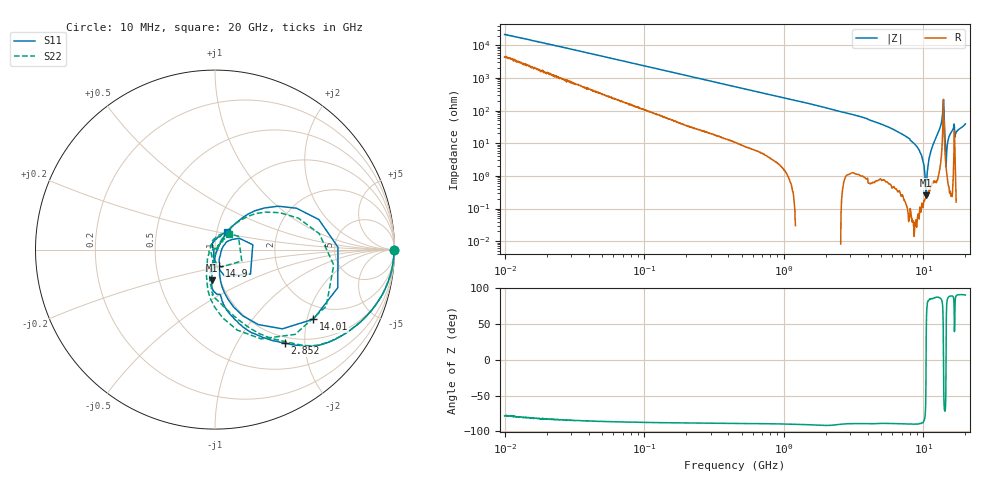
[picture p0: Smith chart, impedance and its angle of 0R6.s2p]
!Keysight Technologies,P5008B,MY61100088,A.16.20.02
!Date: Monday, October 30, 2023 15:55:42
!Correction: S11(C  2-Port  )
!S21(C  2-Port  )
!S12(C  2-Port  )
!S22(C  2-Port  )
!S2P File: Measurements: S11, S21, S12, S22:Log Frequency Sweep
# Hz S  dB  R 50
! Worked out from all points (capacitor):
!   1601 points, 10 MHz to 20 GHz, reference 50 ohm
!   read as one part in series: C = 733 fF near 10.39 MHz
!   lowest |Z| = 253 mohm at 10.43 GHz (marker M1)
!   series resonance near 10.46 GHz, so ESL is about 320 pH
!   S11 on the Smith chart (normalised r, x): 10 MHz: open; 2.852 GHz: 0.90, -1.62; 14.01 GHz: 1.55, -2.19; 14.9 GHz: 1.03, -0.19; 20 GHz: 1.12, +0.22
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1e7  -0.00 -0.3  -46.66 78.1  -46.69 78.9  -0.01 -0.3
3.555162e7  -0.01 -0.9  -36.19 84.1  -36.20 84.3  -0.01 -0.9
1.263918e8  -0.03 -3.2  -25.49 84.5  -25.49 84.5  -0.03 -3.2
4.472136e8  -0.18 -11.0  -14.84 77.8  -14.84 77.9  -0.18 -11.0
1.589917e9  -1.41 -34.7  -5.41 56.2  -5.41 56.2  -1.42 -34.6
2.851944e9  -3.73 -53.2  -2.52 36.7  -2.53 36.7  -3.76 -52.4
5.652411e9  -8.76 -77.3  -0.65 12.1  -0.65 12.1  -8.78 -76.4
1.043228e10  -15.27 -96.1  -0.12 -9.9  -0.12 -9.8  -15.18 -99.7
1.147208e10  -19.32 -96.9  -0.06 -14.1  -0.07 -14.1  -19.07 -101.7
1.214507e10  -27.15 -90.8  -0.03 -17.5  -0.03 -17.4  -27.01 -95.8
1.2437e10  -37.85 -34.3  -0.02 -19.4  -0.03 -19.4  -40.60 -46.6
1.27966e10  -25.10 51.6  -0.06 -22.4  -0.07 -22.4  -25.44 55.6
1.329228e10  -14.89 52.2  -0.32 -29.2  -0.33 -29.2  -15.20 52.8
1.361179e10  -8.85 40.0  -1.21 -39.5  -1.21 -39.5  -9.07 36.5
1.400536e10  -3.46 -35.3  -6.69 11.3  -6.70 11.3  -3.74 -46.6
1.447892e10  -13.55 -79.3  -0.33 -8.9  -0.33 -8.9  -14.07 -102.7
1.489756e10  -20.51 -76.2  -0.06 -16.3  -0.06 -16.3  -21.57 -121.1
1.562236e10  -28.89 -7.8  -0.03 -22.7  -0.03 -22.7  -30.93 145.0
1.653881e10  -16.49 25.0  -0.49 -32.3  -0.49 -32.3  -19.19 58.1
1.750903e10  -39.24 177.7  -0.03 -29.3  -0.03 -29.3  -39.95 177.3
1.792989e10  -32.92 127.4  -0.01 -31.6  -0.01 -31.6  -41.50 49.6
2e10  -18.69 55.4  -0.05 -41.7  -0.05 -41.7  -18.76 48.0
